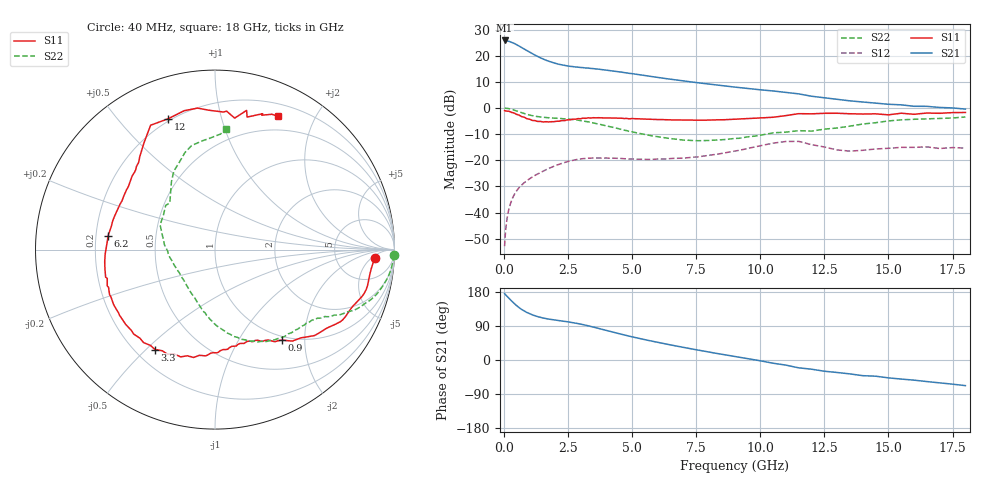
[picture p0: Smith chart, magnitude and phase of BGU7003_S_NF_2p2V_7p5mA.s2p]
!	Filename:	P:\Prog\Test\Noise\ATS_data\Testdata_Net\BGU7002	BGU7003	RN20082092\BGU7003_B1_high	freq_bias	loop_2.2V6.82mA_D.s2p
!	Date/Time:	Tue	16-Sep-08	9:21:42
!	BGU7003_B1_high	freq_bias	loop
!	bias	mode	1:00	Vout=	2.2	"V,"	Iout=	6.935	"mA,"	Vin=	3.353	"V,"	Iin=	0.73	mA
!	Date/time	Sun	Aug	10	20:15:43	2008
!	Device	data	file	deembeded	for	feedlines	and	parallel
!	Original	file:	\BGU7002	BGU7003	RN20082092\BGU7003_B1_high	freq_bias	loop_2.2V6.82mA_R.s2p
!	Feed-files:	PR029V01_high	"frequency_140808_Feed1.s2p,"	PR029V01_high	frequency_140808_Feed2.s2p
!	Parallel-file:	PR029V01_high	frequency_140808_Par.s2p
#	MHz	S	MA	R	50
!	Freq-MHz	S11-mag	S11-arg	S21-mag	S21-arg	S12-mag	S12-arg	S22-mag	S22-arg
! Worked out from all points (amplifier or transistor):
!   152 points, 40 MHz to 18 GHz, reference 50 ohm
!   highest |S21| = 25.8 dB at 40 MHz (marker M1)
!   |S21| within 3 dB of that: start of sweep to 752.9 MHz
!   unconditionally stable (mu >= 1): nowhere
!   at 290 MHz: K = 0.19, MSG = 30.6 dB, |S12| = -35.9 dB
!   at 2.05 GHz: K = 0.56, MSG = 19.5 dB, |S12| = -21.9 dB
!   at 18 GHz: K = 0.68, MSG = 7.4 dB, |S12| = -15.3 dB
!   lowest NFmin = 0.50 dB at 400 MHz
!   S11 on the Smith chart (normalised r, x): 40 MHz: 14, -7; 900 MHz: 0.94, -1.56; 3.3 GHz: 0.28, -0.53; 6.2 GHz: 0.25, +0.06; 12 GHz: 0.19, +0.69; 18 GHz: 0.33, +1.53
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40  0.8911 -3.0  19.6 175.3  0.00228 84.3  0.9966 -1.8
140  0.8731 -11.0  19.21 168.2  0.00795 83.6  0.9857 -6.6
240  0.8548 -18.4  18.63 160.6  0.01341 79.5  0.9636 -11.1
440  0.79 -31.8  16.96 147.4  0.02317 72.9  0.9007 -18.7
550  0.7442 -38.5  15.83 141.1  0.02778 70.2  0.8653 -21.9
650  0.7109 -43.0  14.88 135.8  0.03172 67.9  0.8291 -24.4
900  0.6274 -53.5  12.56 125.7  0.04043 64.0  0.758 -28.8
1100  0.5841 -59.5  11.05 119.5  0.0471 61.9  0.7166 -31.3
1250  0.5703 -63.4  10.13 116.0  0.05233 60.5  0.6955 -33.3
1650  0.5473 -72.9  8.249 109.2  0.0662 56.5  0.6588 -38.0
1950  0.5472 -80.2  7.309 105.8  0.07653 52.7  0.6418 -42.0
2350  0.574 -90.7  6.55 102.1  0.08995 46.6  0.6219 -49.0
3100  0.6402 -114.3  5.926 93.3  0.1078 32.9  0.5669 -65.3
3300  0.6494 -121.0  5.804 90.2  0.1099 29.5  0.5446 -69.7
4700  0.6292 -160.5  4.76 66.1  0.1073 15.0  0.3769 -95.7
6200  0.6003 172.5  3.732 43.9  0.1056 14.9  0.2737 -119.7
7400  0.587 156.6  3.114 28.4  0.1144 16.7  0.2383 -143.1
9200  0.6174 138.4  2.458 7.1  0.156 16.3  0.2641 -178.4
12000  0.7745 109.6  1.681 -24.2  0.1995 -28.6  0.3618 134.1
12500  0.7926 102.5  1.571 -29.6  0.18 -32.7  0.3942 129.0
15500  0.7952 77.2  1.15 -50.3  0.1768 -34.1  0.5936 102.7
18000  0.822 64.7  0.9533 -67.6  0.1717 -47.2  0.6742 84.8
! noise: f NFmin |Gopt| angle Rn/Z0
400  0.504  0.326  8.79  0.131
1000  0.611  0.315  24.58  0.143
1500  0.7  0.307  37.73  0.148
1700  0.736  0.305  43  0.149
2200  0.825  0.301  56.15  0.148
3000  0.968  0.297  77.2  0.141
4400  1.218  0.303  114  0.117
5800  1.467  0.323  150.9  0.093
8000  1.86  0.384  -159.7  0.09
1.2e+04  2.573  0.588  -119.9  0.359
